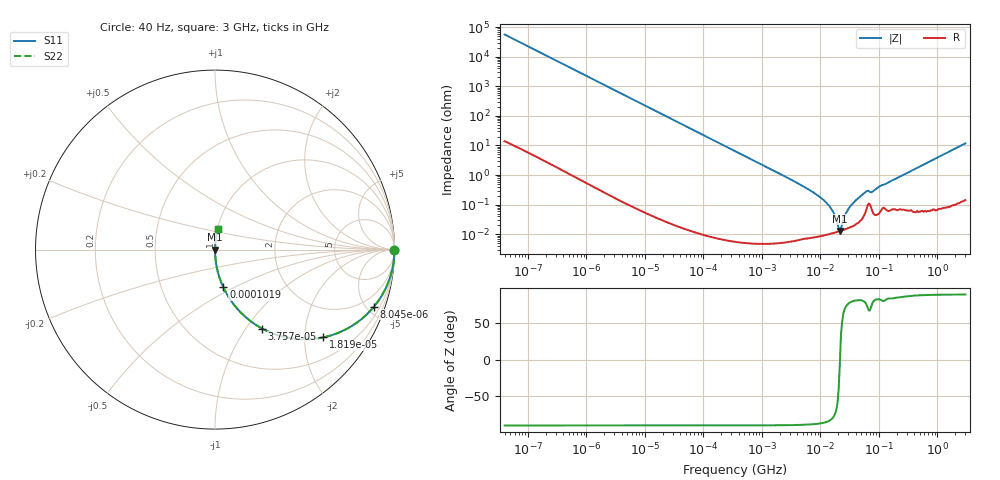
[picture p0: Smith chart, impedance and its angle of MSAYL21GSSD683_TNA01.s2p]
! MSAYL21GSSD683_TNA01  S-PARAMETER MODEL  ( General Type )
! Model Generated by TAIYO YUDEN Corporation (http://www.ty-top.com)
! Version 2.0
! TAIYO YUDEN Control No. 031016
! Copyright(c) 2003 TAIYO YUDEN CO.,LTD. All Rights Reserved.
! Product Description (link to TY-COMPAS)
! https://ds.yuden.co.jp/TYCOMPAS/or/detail?pn=MSAYL21GSSD683KTNA01&u=M
! Products Name : Multilayer Ceramic Capacitors
! Characteristics :
!  Capacitance : 0.068 uF , Rated Voltage : 10V
!  Case Size : 2.0 x 1.25 / 0.079 x 0.049 [mm/inch] , Thickness : 1.25 / 0.049 [mm/inch]
!  (Conditions: Temperature = 25 degC , DC Bias Current/Voltage = 0A / 0V)
! External Node Assignments :
!  1  o---| |---o  2
! GND o---------o GND
! Frequency Range : 40Hz  -  3GHz  [ 401 STEP ]
# MHz S RI R 50
! Freq[MHz].  S11 Real  S11 Imag  S21 Real  S21 Imag  S12 Real  S12 Imag  S22 Real  S22 Imag
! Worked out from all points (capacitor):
!   401 points, 40 Hz to 3 GHz, reference 50 ohm
!   read as one part in series: C = 70.9 nF near 44 Hz
!   lowest |Z| = 12.9 mohm at 21.44 MHz (marker M1)
!   series resonance near 21.56 MHz, so ESL is about 770 pH
!   S11 on the Smith chart (normalised r, x): 40 Hz: open; 8.045 kHz: 1.00, -5.58; 18.19 kHz: 1.00, -2.47; 37.58 kHz: 1.00, -1.19; 101.9 kHz: 1.00, -0.44; 3 GHz: 1.00, +0.23
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4e-05  1 -0.00178  3.62e-06 0.00178  3.62e-06 0.00178  1 -0.00178
0.000834  0.9986 -0.0371  0.00139 0.0371  0.00139 0.0371  0.9986 -0.0371
0.002967  0.9828 -0.1299  0.0172 0.1299  0.0172 0.1299  0.9828 -0.1299
0.008045  0.8861 -0.3176  0.1139 0.3176  0.1139 0.3176  0.8861 -0.3176
0.017386  0.625 -0.484  0.375 0.484  0.375 0.484  0.625 -0.484
0.018193  0.6035 -0.489  0.3965 0.489  0.3965 0.489  0.6035 -0.489
0.037575  0.263 -0.4401  0.737 0.4401  0.737 0.4401  0.263 -0.4401
0.101865  0.0464 -0.2101  0.9536 0.2101  0.9536 0.2101  0.0464 -0.2101
0.362475  0.00387 -0.0617  0.9961 0.0617  0.9961 0.0617  0.00387 -0.0617
7.222098  8.38e-05 -0.00275  0.9999 0.00275  0.9999 0.00275  8.38e-05 -0.00275
10.86056  9.14e-05 -0.00154  0.9999 0.00154  0.9999 0.00154  9.14e-05 -0.00154
14.25536  0.000102 -0.000874  0.9999 0.000874  0.9999 0.000874  0.000102 -0.000874
16.33207  0.000109 -0.000583  0.9999 0.000583  0.9999 0.000583  0.000109 -0.000583
19.57906  0.000121 -0.000203  0.9999 0.000203  0.9999 0.000203  0.000121 -0.000203
21.43715  0.000128 -1.33e-05  0.9999 1.33e-05  0.9999 1.33e-05  0.000128 -1.33e-05
23.47158  0.000136 0.000173  0.9999 -0.000173  0.9999 -0.000173  0.000136 0.000173
29.4429  0.000161 0.000656  0.9998 -0.000656  0.9998 -0.000656  0.000161 0.000656
42.31378  0.000236 0.00152  0.9998 -0.00152  0.9998 -0.00152  0.000236 0.00152
60.81113  0.000678 0.00271  0.9993 -0.00271  0.9993 -0.00271  0.000678 0.00271
76.28187  0.000637 0.00261  0.9994 -0.00261  0.9994 -0.00261  0.000637 0.00261
150.5692  0.00065 0.00586  0.9994 -0.00586  0.9994 -0.00586  0.00065 0.00586
3000  0.0149 0.1154  0.9851 -0.1154  0.9851 -0.1154  0.0149 0.1154
